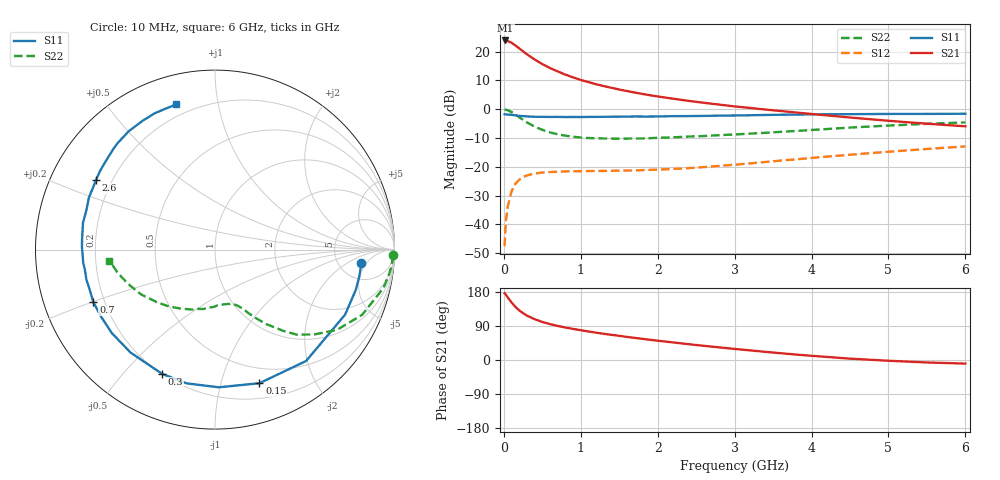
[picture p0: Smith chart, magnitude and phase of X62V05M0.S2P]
! SIEMENS Small Signal Semiconductors
! BFP193W
! Si NPN RF Bipolar Junction Transistor in SOT343
! VCE = 2 V  IC = 5 mA
! Common Emitter S-Parameters:  April 1994
# GHz  S  MA  R  50
!  f  S11  S21  S12  S22
! GHz  MAG  ANG  MAG  ANG  MAG  ANG  MAG  ANG
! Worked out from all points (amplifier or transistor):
!   40 points, 10 MHz to 6 GHz, reference 50 ohm
!   highest |S21| = 23.9 dB at 20 MHz (marker M1)
!   |S21| within 3 dB of that: start of sweep to 212.4 MHz
!   unconditionally stable (mu >= 1): 1.667 GHz to 4.595 GHz
!   at 200 MHz: K = 0.14, MSG = 22.8 dB, |S12| = -24.5 dB
!   at 1.5 GHz: K = 0.93, MSG = 14.1 dB, |S12| = -21.3 dB
!   at 6 GHz: K = 0.94, MSG = 3.5 dB, |S12| = -12.9 dB
!   lowest NFmin = 1.20 dB at 450 MHz
!   S11 on the Smith chart (normalised r, x): 10 MHz: 8.34, -3.77; 150 MHz: 0.34, -1.33; 300 MHz: 0.20, -0.64; 700 MHz: 0.16, -0.20; 2.6 GHz: 0.14, +0.27; 6 GHz: 0.14, +0.76
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0.01  0.8193 -5.2  15.67 176.2  0.0042 88.1  0.994 -1.8
0.02  0.8178 -10.7  15.68 174.1  0.0085 85.2  0.9872 -5.4
0.03  0.8158 -16.1  15.63 171.1  0.0126 82.2  0.9803 -7.8
0.05  0.8103 -26.6  15.35 165.3  0.0203 76.6  0.9629 -12.8
0.1  0.8017 -50.7  14.26 151.9  0.0375 64.9  0.8968 -23.9
0.15  0.7845 -71.6  12.89 140.2  0.0509 54.9  0.8131 -33.4
0.2  0.7675 -88.4  11.43 130.9  0.0598 47.5  0.7287 -40.4
0.25  0.7617 -102.0  10.16 123.5  0.0667 41.4  0.6578 -46.1
0.3  0.7522 -113.1  9.02 117.2  0.071 36.9  0.5927 -49.9
0.4  0.7419 -129.3  7.317 107.7  0.0766 30.3  0.5007 -55.7
0.5  0.7395 -141.0  6.102 100.4  0.0798 26.7  0.4401 -59.5
0.6  0.7365 -149.6  5.197 94.7  0.0815 23.9  0.3975 -62.4
0.7  0.7385 -156.6  4.548 90.0  0.0823 22.5  0.3675 -64.5
0.9  0.7357 -166.9  3.585 82.0  0.0841 20.9  0.3338 -68.5
1.1  0.7379 -174.4  2.969 75.3  0.0847 20.7  0.3167 -72.4
1.6  0.7468 170.9  2.076 60.9  0.0864 23.7  0.3097 -82.8
2.2  0.7601 157.5  1.526 46.4  0.0921 30.0  0.3257 -96.3
2.6  0.7679 149.6  1.297 37.4  0.0992 34.5  0.3431 -105.6
3.2  0.7875 138.8  1.056 25.4  0.1151 39.0  0.3779 -119.3
4.5  0.8231 119.5  0.72 3.6  0.1625 40.8  0.4816 -148.8
5.5  0.8318 109.7  0.562 -6.5  0.2046 37.2  0.5587 -166.9
6  0.8372 105.0  0.506 -9.5  0.2268 34.9  0.592 -174.1
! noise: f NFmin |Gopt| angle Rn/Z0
0.45  1.2  0.26  102  0.14
0.9  1.25  0.38  145  0.12
1.8  2.05  0.56  -161  0.12
